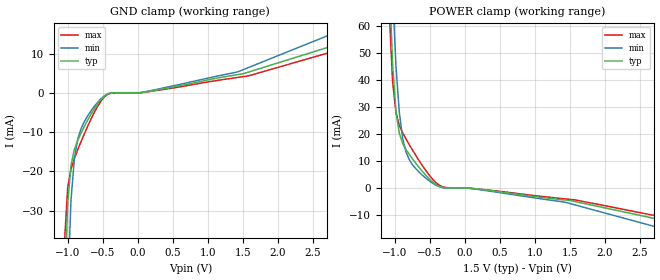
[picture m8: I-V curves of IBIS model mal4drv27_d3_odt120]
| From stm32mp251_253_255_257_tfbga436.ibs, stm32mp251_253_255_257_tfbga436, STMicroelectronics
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[Model] mal4drv27_d3_odt120
Model_type   Input
Polarity   Non-Inverting
Enable   Active-High
C_comp   1.707pF   1.641pF   1.722pF
C_comp_power_clamp   859.437fF   823.771fF   866.710fF
C_comp_gnd_clamp 730.699fF   727.537fF   737.677fF
Vinh = 885.000mV
Vinl = 615.000mV
[Model Spec]
D_overshoot_ampl_h 0.4 NA   NA
D_overshoot_ampl_l 0.4 NA   NA
D_overshoot_area_l 100.000m NA   NA
D_overshoot_area_h 100.000m NA   NA
[Receiver Thresholds]
Vth = 750.000mV
Vth_min = 713.000mV
Vth_max = 788.000mV
Vinh_ac = 135.000mV
Vinh_dc = 100.000mV
Vinl_ac = -135.000mV
Vinl_dc = -100.000mV
Tslew_ac = 5.000ns
Threshold_sensitivity = 0.5
Reference_supply Power_clamp_ref
[Temperature Range]   25.000   125.000   -40.000
[Voltage Range]   1.500V   1.425V   1.575V
[GND Clamp Reference]   0.00V   0.00V   0.00V
[C Comp Corner]
| variable   typ   min   max
C_comp 1.707pF   1.641pF   1.722pF
C_comp_pullup 859.437fF   823.771fF   866.710fF
C_comp_pulldown 730.699fF   727.537fF   737.677fF
[POWER Clamp Reference]   1.500V   1.425V   1.575V
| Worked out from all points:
|   GND clamp passes 1 mA (typ) near -0.49 V on its own axis
|   POWER clamp passes 1 mA (typ) near -0.40 V on its own axis
[GND Clamp]
-1.48V    -1.351A    -1.365A    -1.362A
-1.05V    -54.3mA    -94.78mA   -38.84mA
-1.002V   -28.17mA   -50.17mA   -24.16mA
-954.6mV  -18.46mA   -27.37mA   -19.38mA
-906.8mV  -14.43mA   -16.8mA    -16.71mA
-859.1mV  -12.08mA   -11.81mA   -14.49mA
-715.9mV  -6.877mA   -5.778mA   -8.466mA
-572.7mV  -2.678mA   -2.317mA   -3.337mA
-429.5mV  -188.9uA   -193.5uA   -290.6uA
47.73mV   129.4uA    162.2uA    118.4uA
1.432V    4.741mA    5.468mA    4.022mA
2.959V    13.06mA    16.46mA    11.52mA
[Power Clamp]
-1.459V   564.4mA    584.5mA    561.7mA
-1.077V   76.94mA    109.4mA    64.71mA
-1.03V    45.69mA    72.25mA    39.33mA
-981.8mV  28.14mA    45.14mA    27.8mA
-934.1mV  20.17mA    27.91mA    23.1mA
-886.4mV  16.42mA    18.3mA     20.36mA
-838.6mV  14.12mA    13.22mA    18.08mA
-695.5mV  8.945mA    6.973mA    11.84mA
-409.1mV  1.173mA    923.6uA    1.848mA
-265.9mV  -15.52uA   -111.5uA   43.5uA
1.405V    -4.456mA   -5.248mA   -4.062mA
2.98V     -12.88mA   -16.27mA   -11.67mA
